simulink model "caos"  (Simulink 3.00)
settings: Solver=ode45  StartTime=0.0  StopTime=50  MaxStep=0.01  RelTol=1e-5  AbsTol=1e-5

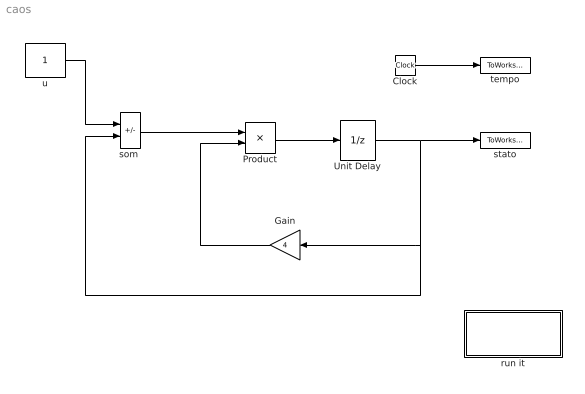
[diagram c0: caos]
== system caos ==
  Clock : Clock
  Gain : Gain  Orientation=left  Gain=4  SaturateOnIntegerOverflow=on
  Product : Product  Inputs=2  SaturateOnIntegerOverflow=on
  Unit Delay : UnitDelay  X0=0.75  SampleTime=1
  run it : Subsystem  Description=plot
  "som " : Sum  Inputs=+-  SaturateOnIntegerOverflow=on
  stato : ToWorkspace  VariableName=x  SampleTime=1  SaveFormat=Matrix
  tempo : ToWorkspace  VariableName=k  SampleTime=1  SaveFormat=Matrix
  u : Constant  Value=1
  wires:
  Product/1 -> Unit Delay/1
  u/1 -> "som "/1
  "som "/1 -> Product/1
  Unit Delay/1 -> Gain/1, "som "/2, stato/1
  Gain/1 -> Product/2
  Clock/1 -> tempo/1

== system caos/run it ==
